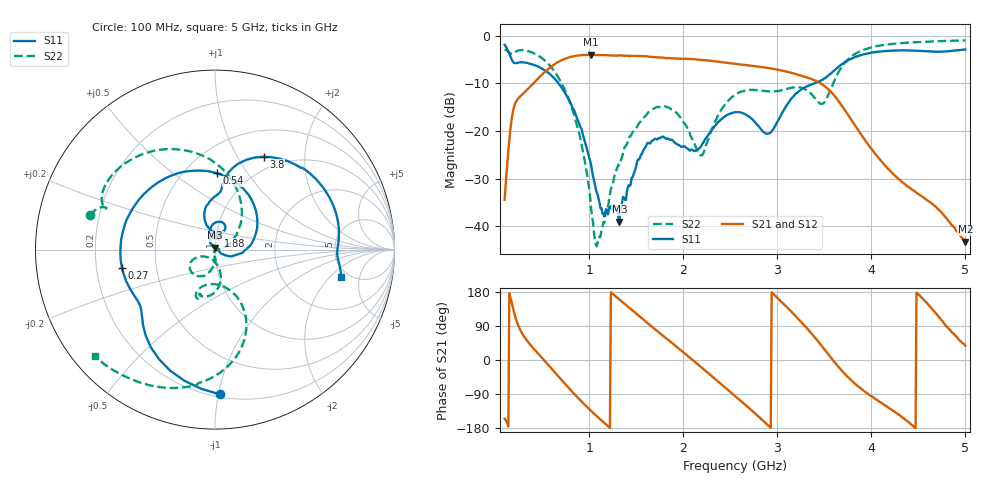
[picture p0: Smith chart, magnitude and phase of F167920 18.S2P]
!  2-Port S-parameters saved by WinCal
! VAR MeasName=S-Parameters (CALIBRATED_DATA) read from VNA (N5242A)
! VAR MeasDate=2016-11-22 9:56:04
! VAR NAME=F167920 18
! VAR FILENAME=F167920 18.S2P
! VAR DATE=2016-11-22 9:56:04
! VAR PHYS_PORTS=1,2
# Hz S DB R 50
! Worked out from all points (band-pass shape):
!   491 points, 100 MHz to 5 GHz, reference 50 ohm
!   highest |S21| = -3.98 dB at 1.02 GHz (marker M1); lowest = -43.3 dB at 5 GHz (marker M2)
!   |S21| within 3 dB of the highest: 564.4 MHz to 2.966 GHz (2.401 GHz wide, 136 % of centre)
!   lowest |S11| = -39.0 dB at 1.32 GHz (marker M3), VSWR 1.02, Z = 50 + j1.12 ohm
!   |S11| at or under -10 dB: 673.8 MHz to 3.393 GHz (2.719 GHz wide, 134 % of centre)
!   |S22| runs from -44.2 to -1.0 dB; largest |S21 - S12| = 0.00099
!   S11 on the Smith chart (normalised r, x): 100 MHz: 0.22, -1.01; 270 MHz: 0.31, -0.09; 540 MHz: 0.71, +0.73; 1.88 GHz: 1.03, +0.16; 3.8 GHz: 0.83, +1.30; 5 GHz: 4.30, -2.75
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1e8  -1.87 -88.1  -34.45 -154.8  -34.43 -154.1  -2.82 164.6
1.8e8  -5.15 -137.4  -16.86 146.7  -16.87 146.7  -3.79 159.3
2.7e8  -5.54 -169.1  -12.63 77.4  -12.63 77.4  -2.99 149.3
4.1e8  -6.10 135.0  -9.91 29.7  -9.91 29.7  -3.64 124.5
5.4e8  -7.43 88.7  -7.39 -6.3  -7.39 -6.3  -5.39 99.4
7e8  -10.69 36.3  -5.17 -51.1  -5.18 -51.1  -9.73 65.3
9.2e8  -19.67 -21.1  -4.02 -109.9  -4.02 -109.8  -23.14 16.9
1.02e9  -27.14 -32.4  -3.98 -134.4  -3.98 -134.4  -36.25 -3.9
1.09e9  -33.41 -14.6  -4.03 -150.4  -4.03 -150.4  -43.36 -80.0
1.32e9  -39.04 89.6  -4.10 160.2  -4.10 160.2  -27.21 -93.4
1.53e9  -25.98 120.5  -4.25 116.2  -4.25 116.2  -18.33 -102.0
1.74e9  -21.45 91.6  -4.53 73.0  -4.53 72.9  -14.93 -128.3
1.88e9  -21.89 76.5  -4.71 44.9  -4.71 44.9  -15.52 -146.3
2.19e9  -23.14 101.8  -5.06 -19.0  -5.06 -19.0  -25.15 -116.6
2.55e9  -16.03 81.3  -5.88 -94.6  -5.89 -94.6  -12.40 -90.9
2.94e9  -20.11 95.2  -6.88 178.6  -6.89 178.5  -11.70 -108.7
3.17e9  -12.73 103.7  -7.86 122.5  -7.87 122.4  -10.85 -107.8
3.37e9  -10.15 86.8  -9.12 68.1  -9.13 68.2  -12.40 -112.4
3.49e9  -9.11 83.6  -10.37 31.7  -10.39 31.7  -14.17 -85.7
3.8e9  -4.67 62.2  -18.05 -56.7  -18.08 -56.7  -4.14 -80.1
4.19e9  -3.14 27.6  -28.19 -127.2  -28.24 -126.8  -1.76 -109.5
5e9  -2.86 -12.4  -43.29 37.6  -43.19 38.4  -0.96 -138.4
